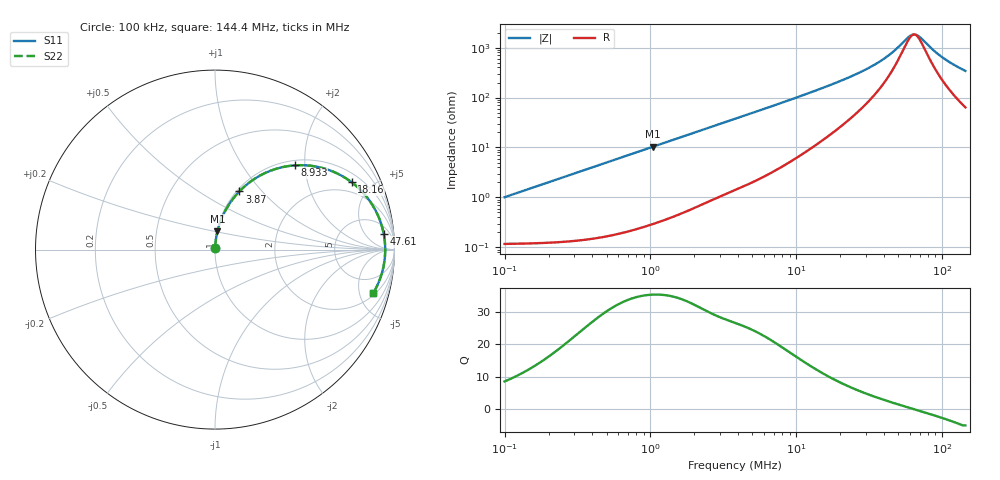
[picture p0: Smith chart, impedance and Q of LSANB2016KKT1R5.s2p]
! LSANB2016KKT1R5  S-PARAMETER MODEL  ( General Type )
! Model Generated by TAIYO YUDEN Corporation (http://www.ty-top.com)
! Version 3.0
! TAIYO YUDEN Control No. 20210629
! Copyright(c) 2013 TAIYO YUDEN CO.,LTD. All Rights Reserved.
! Product Description (link to TY-COMPAS)
! https://ds.yuden.co.jp/TYCOMPAS/or/detail?pn=LSANB2016KKT1R5M&u=M
! Products Name : Inductors
! Characteristics :
!  Inductance : 1.5 uH , SRF(min) : -Hz , DC Resistance(max) : 0.13 Ohm
!  Rated Current : Saturation :1600 mA , Temp Rise : 1650 mA (40 degC)
!  Case Size : 2.0 x 1.6 / 0.079 x 0.063 [mm/inch] , Thickness : 1 / 0.039 [mm/inch]
!  (Conditions: Temperature = 25 degC , DC Bias Current/Voltage = 0A / 0V)
! External Node Assignments :
!  1  o---GGG---o  2
! GND o---------o GND
! Frequency Range : 0.1MHz  -  144.390904MHz  [ 402 STEP ]
# MHz S RI R 50
! Freq[MHz].  S11 Real  S11 Imag  S21 Real  S21 Imag  S12 Real  S12 Imag  S22 Real  S22 Imag
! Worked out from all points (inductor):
!   401 points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, 100 kHz to 144.4 MHz, reference 50 ohm
!   read as one part in series: L = 1.6 uH near 103.7 kHz
!   highest Q = 35.4 at 1.045 MHz (marker M1), where L = 1.59 uH
!   self-resonance near 64.3 MHz
!   S11 on the Smith chart (normalised r, x): 100 kHz: 1.00, +0.02; 3.87 MHz: 1.03, +0.76; 8.933 MHz: 1.10, +1.77; 18.16 MHz: 1.41, +3.80; 47.61 MHz: 10, +16; 144.4 MHz: 2.27, -6.71
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0.1  0.00127 0.01  0.9987 -0.01  0.9987 -0.01  0.00127 0.01
0.338238  0.00254 0.0338  0.9975 -0.0338  0.9975 -0.0338  0.00254 0.0338
1.044604  0.0136 0.1024  0.9864 -0.1024  0.9864 -0.1024  0.0136 0.1024
1.144052  0.0159 0.1118  0.9841 -0.1118  0.9841 -0.1118  0.0159 0.1118
2.283506  0.0548 0.2119  0.9452 -0.2119  0.9452 -0.2119  0.0548 0.2119
3.869624  0.1356 0.3241  0.8644 -0.3241  0.8644 -0.3241  0.1356 0.3241
5.773557  0.2531 0.4136  0.7469 -0.4136  0.7469 -0.4136  0.2531 0.4136
8.933381  0.4432 0.4692  0.5568 -0.4692  0.5568 -0.4692  0.4432 0.4692
12.85266  0.6194 0.4486  0.3806 -0.4486  0.3806 -0.4486  0.6194 0.4486
18.15812  0.7616 0.3752  0.2384 -0.3752  0.2384 -0.3752  0.7616 0.3752
30.21613  0.8915 0.2238  0.1085 -0.2238  0.1085 -0.2238  0.8915 0.2238
36.90848  0.9192 0.1626  0.0808 -0.1626  0.0808 -0.1626  0.9192 0.1626
43.47261  0.9343 0.1137  0.0657 -0.1137  0.0657 -0.1137  0.9343 0.1137
47.6113  0.9401 0.0869  0.0599 -0.0869  0.0599 -0.0869  0.9401 0.0869
59.22379  0.9477 0.0236  0.0523 -0.0236  0.0523 -0.0236  0.9477 0.0236
62.54502  0.9482 0.00795  0.0518 -0.00795  0.0518 -0.00795  0.9482 0.00795
66.05251  0.9483 -0.00773  0.0517 0.00773  0.0517 0.00773  0.9483 -0.00773
71.03701  0.9475 -0.0287  0.0525 0.0287  0.0525 0.0287  0.9475 -0.0287
86.77049  0.9404 -0.0867  0.0596 0.0867  0.0596 0.0867  0.9404 -0.0867
100.3605  0.9303 -0.1297  0.0697 0.1297  0.0697 0.1297  0.9303 -0.1297
120.3792  0.9109 -0.1847  0.0891 0.1847  0.0891 0.1847  0.9109 -0.1847
144.3909  0.8827 -0.2408  0.1173 0.2408  0.1173 0.2408  0.8827 -0.2408
